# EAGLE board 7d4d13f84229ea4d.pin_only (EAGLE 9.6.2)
REV: B

Size 65 x 30.7 mm. Coordinates in mm from the lower left corner, seen from the top.
Outline: 0,19.56 0,19.68
Outline: 0,27.7 0,3 arc90 3,0 62,0 arc90 65,3 65,27.7 arc90 62,30.7 3,30.7 arc90 0,27.7
Copper layers (1*16): Top 0.035mm / dielectric 1.5mm / Bottom 0.035mm
Design rules "adafruit *": minimum track width 8mil, minimum drill 15.5mil, track to track 8mil, track to pad 8mil, pad to pad 8mil, via to via 8mil, smd to smd 8mil, copper to edge 10mil, drill to drill 8mil, minimum pad ring 10mil, minimum via ring 8mil, stop-mask expansion 2mil, vias tented up to drill 20mil, thermal gap 10mil

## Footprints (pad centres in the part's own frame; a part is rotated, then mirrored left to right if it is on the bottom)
SOLDERJUMPER_REFLOW_NOPASTE = smd 1.168 x 1.6: 1 -0.762,0; 2 0.762,0
0603-NO = smd 1.075 x 1: 1 -0.85,0; 2 0.85,0
PANASONIC_C = smd 2.6 x 1.4: + 2.05,0; - -2.05,0
0805-NO = smd 1.24 x 1.5: 1 -0.95,0; 2 0.95,0
1X25_ROUND_70MIL = drill 1 pad 1.676: 1 -30.48,0; 2 -27.94,0; 3 -25.4,0; 4 -22.86,0; 5 -20.32,0; 6 -17.78,0; 7 -15.24,0; 8 -12.7,0; 9 -10.16,0; 10 -7.62,0; 11 -5.08,0; 12 -2.54,0; 13 0,0; 14 2.54,0; 15 5.08,0; 16 7.62,0; 17 10.16,0; 18 12.7,0; 19 15.24,0; 20 17.78,0; 21 20.32,0; 22 22.86,0; 23 25.4,0; 24 27.94,0; 25 30.48,0
JST_SH4 = smd 0.6 x 1.55: 1 -1.5,2.006; 2 -0.5,2.006; 3 0.5,2.006; 4 1.5,2.006 | smd 1.2 x 1.8: MT1 -2.8,-1.894; MT2 2.8,-1.894
FIDUCIAL_1MM = smd 1 x 1: 1 0,0
SSOP24 = smd 0.4 x 1.25: 1 -3.575,-3.625; 2 -2.925,-3.625; 3 -2.275,-3.625; 4 -1.625,-3.625; 5 -0.975,-3.625; 6 -0.325,-3.625; 7 0.325,-3.625; 8 0.975,-3.625; 9 1.625,-3.625; 10 2.275,-3.625; 11 2.925,-3.625; 12 3.575,-3.625; 13 3.575,3.625; 14 2.925,3.625; 15 2.275,3.625; 16 1.625,3.625; 17 0.975,3.625; 18 0.325,3.625; 19 -0.325,3.625; 20 -0.975,3.625; 21 -1.625,3.625; 22 -2.275,3.625; 23 -2.925,3.625; 24 -3.575,3.625
1X04_ROUND = drill 1 pad 1.778: 1 -3.81,0; 2 -1.27,0; 3 1.27,0; 4 3.81,0
CHIPLED_0805_NOOUTLINE = smd 1.2 x 1.2: A 0,-1.05; C 0,1.05
TERMBLOCK_1X2-3.5MM = drill 1 pad 2.184: 1 1.8,0; 2 -1.7,0
D-PAK_TO252AA = smd 1 x 1.6: 1 -2.28,-4.8; 3 2.28,-4.8 | smd 5.4 x 6.2: 4 0,2.5
RESPACK_4X0603 = smd 0.45 x 0.9: 1 -1.3,-0.85; 2 -0.4,-0.85; 3 0.4,-0.85; 4 1.3,-0.85; 5 1.3,0.85; 6 0.4,0.85; 7 -0.4,0.85; 8 -1.3,0.85
PI_BONNET_THMSMT = drill 0.9 pad 1.27: 1 -24.13,-1.27; 2 -24.13,1.27; 3 -21.59,-1.27; 4 -21.59,1.27; 37 21.59,-1.27; 38 21.59,1.27; 39 24.13,-1.27; 40 24.13,1.27 | drill 0.9 pad 1.676: 5 -19.05,-1.27; 6 -19.05,1.27; 7 -16.51,-1.27; 8 -16.51,1.27; 9 -13.97,-1.27; 10 -13.97,1.27; 11 -11.43,-1.27; 12 -11.43,1.27; 13 -8.89,-1.27; 14 -8.89,1.27; 15 -6.35,-1.27; 16 -6.35,1.27; 17 -3.81,-1.27; 18 -3.81,1.27; 19 -1.27,-1.27; 20 -1.27,1.27; 21 1.27,-1.27; 22 1.27,1.27; 23 3.81,-1.27; 24 3.81,1.27; 25 6.35,-1.27; 26 6.35,1.27; 27 8.89,-1.27; 28 8.89,1.27; 29 11.43,-1.27; 30 11.43,1.27; 31 13.97,-1.27; 32 13.97,1.27; 33 16.51,-1.27; 34 16.51,1.27; 35 19.05,-1.27; 36 19.05,1.27 | smd 1 x 1 bottom: 41 -29.96,2.71; 42 29.73,2.71 | smd 1.524 x 2.286 bottom: S1 -24.13,-2.542; S2 -24.13,2.538; S3 -21.59,-2.542; S4 -21.59,2.538; S37 21.59,-2.542; S38 21.59,2.538; S39 24.13,-2.542; S40 24.13,2.538 | smd 1.524 x 2.54 bottom: S5 -19.05,-2.415 | smd 1.524 x 3.048 bottom: S6 -19.05,2.157; S7 -16.51,-2.161; S8 -16.51,2.157; S9 -13.97,-2.161; S10 -13.97,2.157; S11 -11.43,-2.161; S12 -11.43,2.157; S13 -8.89,-2.161; S14 -8.89,2.157; S15 -6.35,-2.161; S16 -6.35,2.157; S17 -3.81,-2.161; S18 -3.81,2.157; S19 -1.27,-2.161; S20 -1.27,2.157; S21 1.27,-2.161; S22 1.27,2.157; S23 3.81,-2.161; S24 3.81,2.157; S25 6.35,-2.161; S26 6.35,2.157; S27 8.89,-2.161; S28 8.89,2.157; S29 11.43,-2.161; S30 11.43,2.157; S31 13.97,-2.161; S32 13.97,2.157; S33 16.51,-2.161; S34 16.51,2.157; S35 19.05,-2.161; S36 19.05,2.157 | hole 2.8: -29,0; 29,0; 29,-23; -29,-23 | hole 2: -22.86,0; 22.86,0
TSSOP28 = smd 0.305 x 0.991: 1 -4.225,-2.918; 2 -3.575,-2.918; 3 -2.925,-2.918; 4 -2.275,-2.918; 5 -1.625,-2.918; 6 -0.975,-2.918; 7 -0.325,-2.918; 8 0.325,-2.918; 9 0.975,-2.918; 10 1.625,-2.918; 11 2.275,-2.918; 12 2.925,-2.918; 13 3.575,-2.918; 14 4.225,-2.918; 15 4.225,2.918; 16 3.575,2.918; 17 2.925,2.918; 18 2.275,2.918; 19 1.625,2.918; 20 0.975,2.918; 21 0.325,2.918; 22 -0.325,2.918; 23 -0.975,2.918; 24 -1.625,2.918; 25 -2.275,2.918; 26 -2.925,2.918; 27 -3.575,2.918; 28 -4.225,2.918
TERMBLOCK_1X3-3.5MM = drill 1 pad 2.184: 1 3.5,0; 2 0,0; 3 -3.5,0

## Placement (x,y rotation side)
A0  [SOLDERJUMPER_REFLOW_NOPASTE]  24.51,8.64 90 bottom
A1  [SOLDERJUMPER_REFLOW_NOPASTE]  27.05,8.64 90 bottom
A2  [SOLDERJUMPER_REFLOW_NOPASTE]  29.59,8.64 90 bottom
A3  [SOLDERJUMPER_REFLOW_NOPASTE]  32.13,8.64 270 bottom
A4  [SOLDERJUMPER_REFLOW_NOPASTE]  34.92,8.64 270 bottom
C1  0.1uF  [0603-NO]  17.78,10.29 0 top
C3  0.1uF  [0603-NO]  25.78,8.38 0 top
C4  47uF/16v  [PANASONIC_C]  46.1,15.62 180 top
C5  47uF+/16v  [PANASONIC_C]  17.02,15.11 90 top
C6  10uF  [0805-NO]  43.56,11.05 270 top
C10  10uF  [0805-NO]  14.86,10.54 270 top
CONN1  HEADER-1X25  [1X25_ROUND_70MIL]  32.77,21.21 0 top
CONN2  STEMMA_I2C_QT  [JST_SH4]  61.8,15.1 90 top
FID1  FIDUCIAL_1MM  [FIDUCIAL_1MM]  2.79,29.21 0 top
FID2  FIDUCIAL_1MM  [FIDUCIAL_1MM]  64.01,3.68 0 top
FID3  FIDUCIAL_1MM  [FIDUCIAL_1MM]  1.02,3.81 0 top
IC1  TB6612FNG  [SSOP24]  9.27,13.84 0 top
IC3  TB6612FNG  [SSOP24]  37.97,14.1 0 top
JP1  [1X04_ROUND]  2.67,12.95 90 top
LED1  Green  [CHIPLED_0805_NOOUTLINE]  45.47,2.03 180 top
MPOWER  1x2 3.5mm  [TERMBLOCK_1X2-3.5MM]  53.09,3.68 0 top
PLABEL0  [PLABEL0]  2.41,19.3 0 top
PLABEL1  [PLABEL1]  4.83,22.86 0 top
PLABEL2  [PLABEL2]  7.49,19.3 0 top
PLABEL3  [PLABEL3]  10.03,22.86 0 top
PLABEL4  [PLABEL4]  12.45,19.3 0 top
PLABEL5  [PLABEL5]  14.99,22.86 0 top
PLABEL6  [PLABEL6]  17.53,19.3 0 top
PLABEL7  [PLABEL7]  20.19,22.99 0 top
PLABEL8  [PLABEL8]  22.48,19.3 0 top
PLABEL9  [PLABEL9]  24.89,22.99 0 top
PLABEL10  [PLABEL10]  27.43,19.3 0 top
PLABEL11  [PLABEL11]  30.1,22.99 0 top
PLABEL12  [PLABEL12]  32.77,19.43 0 top
PLABEL13  [PLABEL13]  35.31,22.99 0 top
PLABEL14  [PLABEL14]  37.85,19.3 0 top
PLABEL15  [PLABEL15]  40.39,22.99 0 top
PLABEL16  [PLABEL16]  42.93,19.3 0 top
PLABEL17  [PLABEL17]  45.47,22.99 0 top
PLABEL18  [PLABEL18]  48.01,19.3 0 top
PLABEL19  [PLABEL19]  50.29,22.99 0 top
PLABEL20  [PLABEL20]  52.96,19.43 0 top
PLABEL21  [PLABEL21]  55.37,22.99 0 top
PLABEL22  [PLABEL22]  57.91,19.43 0 top
PLABEL23  [PLABEL23]  60.45,22.99 0 top
PLABEL24  [PLABEL24]  63.25,19.3 0 top
PLABEL25  [PLABEL25]  58.45,12.53 90 top
PLABEL26  [PLABEL26]  8.83,7.57 0 top
PLABEL27  [PLABEL27]  19.49,7.57 0 top
PLABEL28  [PLABEL28]  14.01,7.46 0 top
PLABEL29  [PLABEL29]  38.06,7.44 0 top
PLABEL30  [PLABEL30]  27.72,7.54 0 top
PLABEL31  [PLABEL31]  32.88,7.62 0 top
PLABEL33  [PLABEL33]  44.38,6.38 0 top
PLABEL34  [PLABEL34]  47.35,0.89 0 top
PLABEL35  [PLABEL35]  57.5,0.68 0 top
PLABEL36  [PLABEL36]  1.14,15.75 90 top
PLABEL37  [PLABEL37]  1.14,13.34 90 top
PLABEL38  [PLABEL38]  1.14,10.54 90 top
PLABEL39  [PLABEL39]  1.14,7.86 90 top
PLABEL40  [PLABEL40]  2.67,6.25 0 top
PLABEL41  [PLABEL41]  24.26,11.56 90 bottom
PLABEL42  [PLABEL42]  27,11.56 90 bottom
PLABEL43  [PLABEL43]  29.64,11.56 90 bottom
PLABEL44  [PLABEL44]  32.08,11.56 90 bottom
PLABEL45  [PLABEL45]  34.97,11.56 90 bottom
PLABEL46  [PLABEL46]  29.59,6.22 0 bottom
PLABEL47  [PLABEL47]  57.53,5.21 0 top
Q1  AOD417  [D-PAK_TO252AA]  52.96,13.72 180 top
R1  10K Pack  [RESPACK_4X0603]  31.37,11.43 90 top
R2  10K  [0603-NO]  31.37,14.22 180 top
R7  1K  [0603-NO]  45.47,10.92 90 top
RPI1  RASPBERRYPI_BPLUS_BONNET_THMSMT  [PI_BONNET_THMSMT]  32.5,26.5 0 top
U2  PCA9685  [TSSOP28]  25.65,13.97 90 top
U$6  [PCBFEAT-REV-040]  5.59,1.61 0 top
U$8  [ADAFRUIT_TEXT_20MM]  60.45,8.76 0 bottom
U$14  [ADAFRUIT_3.5MM]  29.6,14.9 0 top
U$15  [STEMMAQT]  61.98,9.78 90 bottom
X1  1x2 3.5mm  [TERMBLOCK_1X2-3.5MM]  39.9,3.7 0 top
X2  1x2 3.5mm  [TERMBLOCK_1X2-3.5MM]  21.2,3.7 0 top
X3  1x3 3.5mm  [TERMBLOCK_1X3-3.5MM]  31.2,3.7 0 top
X4  1x3 3.5mm  [TERMBLOCK_1X3-3.5MM]  12.5,3.7 0 top

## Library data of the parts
A0 A1-A4 C1 C3 C6 C10 CONN1 JP1 R1 R2 R7 U2 U$6 U$8 U$14 = microbuilder
C4 C5 = microbuilder; ROT: 180
CONN2 = adafruit_electromech; LCSC: C2905006
FID1-FID3 = microbuilder; BOM: EXCLUDE
IC1 IC3 = adafruit
LED1 = microbuilder; ROT: 270
MPOWER X1 X2 = adafruit_electromech; FORCETHM: 1; ROT: 0
PLABEL0 PLABEL1-PLABEL31 PLABEL33-PLABEL47 = pinguin
Q1 = transistor-power
RPI1 = adafruit_sbc
U$15 = silks
X3 X4 = adafruit_electromech; FORCETHM: 1

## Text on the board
Pinguin_tBackup: SCL | RXD | #17 | #27 | #23 | #25 | MISO | CE0 | #5 | #12 | #16 | #20 | SDA | TXD | #4 | #18 | #22 | #24 | MOSI | CLK | CE1 | #6 | #13 | #19 | #21 | 15 | adafruit! | 14 | #1 | M1 | GND | M2 | M3 | GND | M4 | #0 | extra / PWM | 5-12V / Motor / Power | DC & / Stepper / Motor / Bonnet | + | -
Pinguin_bBackup: A0 | A1 | A2 | A3 | A4 | I2C Address

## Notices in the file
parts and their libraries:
microbuilder: This work is placed in the public domain, and may be freely used for commercial and non-commercial work with the following conditions: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
